DATA_BLOCK DB 1
STRUCT
	Value		: INT
END_STRUCT
BEGIN
	Value		:= 8290
END_DATA_BLOCK


FUNCTION_BLOCK FB 1
BEGIN
	L		W#16#4321
	T		MW 0
END_FUNCTION_BLOCK


FUNCTION FC 1 : VOID
BEGIN
	L		W#16#1234
	T		MW 0
	CALL		FC 2
END_FUNCTION


FUNCTION FC 2 : VOID
BEGIN
	L		W#16#6789
	T		MW 0
	L		10
	T		LB 0
END_FUNCTION


FUNCTION FC 3 : VOID
BEGIN
	L		1
	T		LB 0
	CALL		FC 2
	__ASSERT==	LB 0,	1
END_FUNCTION


FUNCTION FC 4 : VOID
VAR_INPUT
	INPVAR		: INT
END_VAR
BEGIN
	L		#INPVAR
	__ASSERT==	__ACCU 1,	9976
END_FUNCTION


FUNCTION FC 5 : VOID
VAR_INPUT
	INPVAR2		: INT
END_VAR
BEGIN
	CALL FC 4 (
		INPVAR		:= #INPVAR2,	// This is a parameter
	)
END_FUNCTION


FUNCTION FC 6 : VOID
BEGIN
	// Only check OV and OS bits
	__ASSERT==	__STW OV,	1
	__ASSERT==	__STW OS,	0
	L		1
	L		1
	+I
	__ASSERT==	__STW OV,	0
	__ASSERT==	__STW OS,	0
END_FUNCTION


FUNCTION FC 7 : VOID
BEGIN
	// Trigger an overflow
	__ASSERT==	__STW OV,	0
	__ASSERT==	__STW OS,	0
	L		30000
	L		30000
	+I
	__ASSERT==	__STW OV,	1
	__ASSERT==	__STW OS,	1
END_FUNCTION


FUNCTION_BLOCK FB 10
VAR_INPUT
	INVAR1		: DWORD
	INVAR2		: INT
	//TODO more
END_VAR
VAR_OUTPUT
	RETURNVALUE	: INT
END_VAR
BEGIN
	L		#INVAR1
	__ASSERT==	__ACCU 1,	DW#16#88776655
	CALL FC 10 (
		INPUTVAR1	:= #INVAR1,
		INPUTVAR2	:= #INVAR2,
		INVAR_DB	:= DB1.DBW 0,
		RET_VAL		:= #RETURNVALUE,
	)
END_FUNCTION_BLOCK


DATA_BLOCK DB 10
FB 10
BEGIN
END_DATA_BLOCK


FUNCTION FC 10 : INT
VAR_INPUT
	INPUTVAR1	: DWORD
	INPUTVAR2	: INT
	INVAR_DB	: INT
	//TODO more
END_VAR
BEGIN
	L		#INPUTVAR1
	__ASSERT==	__ACCU 1,	DW#16#88776655
	L		P##INPUTVAR1
	UD		DW#16#FFF80000
	__ASSERT==	__ACCU 1,	DW#16#84000000

	L		#INPUTVAR2
	__ASSERT==	__ACCU 1,	8290

	L		#INVAR_DB
	__ASSERT==	__ACCU 1,	8290

	L		99
	T		#RET_VAL
	L		#RET_VAL
	__ASSERT==	__ACCU 1,	99
	L		P##RET_VAL
	UD		DW#16#FFF80000
	__ASSERT==	__ACCU 1,	DW#16#84000000

	CALL FC 11 (
		IN1	:= #INVAR_DB,
	)
END_FUNCTION


FUNCTION FC 11 : VOID
VAR_INPUT
	IN1		: INT
END_VAR
BEGIN
	L		#IN1
	__ASSERT==	__ACCU 1,	8290
END_FUNCTION


ORGANIZATION_BLOCK OB 1
BEGIN
	CALL		FC 1
	__ASSERT==	MW 0,	W#16#6789
	L		0
	T		MW 0
	__ASSERT==	MW 0,	0
	UC		FC 1
	__ASSERT==	MW 0,	W#16#6789
	L		0
	T		MW 0
	__ASSERT==	MW 0,	0
	SET
	CC		FC 1
	__ASSERT==	MW 0,	W#16#6789
	L		0
	T		MW 0
	__ASSERT==	MW 0,	0
	CLR
	CC		FC 1
	__ASSERT==	MW 0,	0

	// Test localdata stack
	L		255
	T		LB 0
	__ASSERT==	LB 0,	255
	CALL		FC 3
	__ASSERT==	LB 0,	255

	CALL FC 5 (
		INPVAR2		:= 9976,
	)

	// Test OV/OS bits over call boundaries
	__STWRST
	L		30000
	L		30000
	+I
	__ASSERT==	__STW OV,	1
	__ASSERT==	__STW OS,	1
	CALL FC 6
	__ASSERT==	__STW OV,	0
	__ASSERT==	__STW OS,	0
	__STWRST
	CALL FC 7
	__ASSERT==	__STW OV,	1
	__ASSERT==	__STW OS,	0


	// Test raw FB call
	L		0
	T		MW 0
	CLR
	UC		FB 1
	L		MW 0
	__ASSERT==	__ACCU 1,	W#16#4321
	L		0
	T		MW 0
	SET
	CC		FB 1
	L		MW 0
	__ASSERT==	__ACCU 1,	W#16#4321


	// Test indirect calls
	L		0
	T		MW 0
	L		1
	T		MW 50
	CLR
	UC		FC [MW 50]
	L		MW 0
	__ASSERT==	__ACCU 1,	W#16#6789
	L		0
	T		MW 0
	SET
	CC		FC [MW 50]
	L		MW 0
	__ASSERT==	__ACCU 1,	W#16#6789
	L		0
	T		MW 0
	CLR
	UC		FB [MW 50]
	L		MW 0
	__ASSERT==	__ACCU 1,	W#16#4321
	L		0
	T		MW 0
	SET
	CC		FB [MW 50]
	L		MW 0
	__ASSERT==	__ACCU 1,	W#16#4321


	// Test parameter forwarding (FB->FC)
	CALL FB 10, DB 10 (
		INVAR1		:= DW#16#88776655,
		INVAR2		:= DB1.DBW 0,
		RETURNVALUE	:= MW 0,
	)
	L		MW 0
	__ASSERT==	__ACCU 1,	99

END_ORGANIZATION_BLOCK
